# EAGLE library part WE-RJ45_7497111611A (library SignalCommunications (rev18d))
Order Code 7497111611A Design THT xBase-T 10/100/1000 Base-T Ports 1x1 + 2xUSB Application Standard USB2.0 Tab Position UP LED (Left-Right) GREEN/ORANGE-YELLOW EMI Fingers YES Details see: http://katalog.we-online.de/en/pbs/WE-LAN_RJ45/7497111611A? Updated by Yingchun Shan 2016-08-23 2014 (C) Würth Elektronik
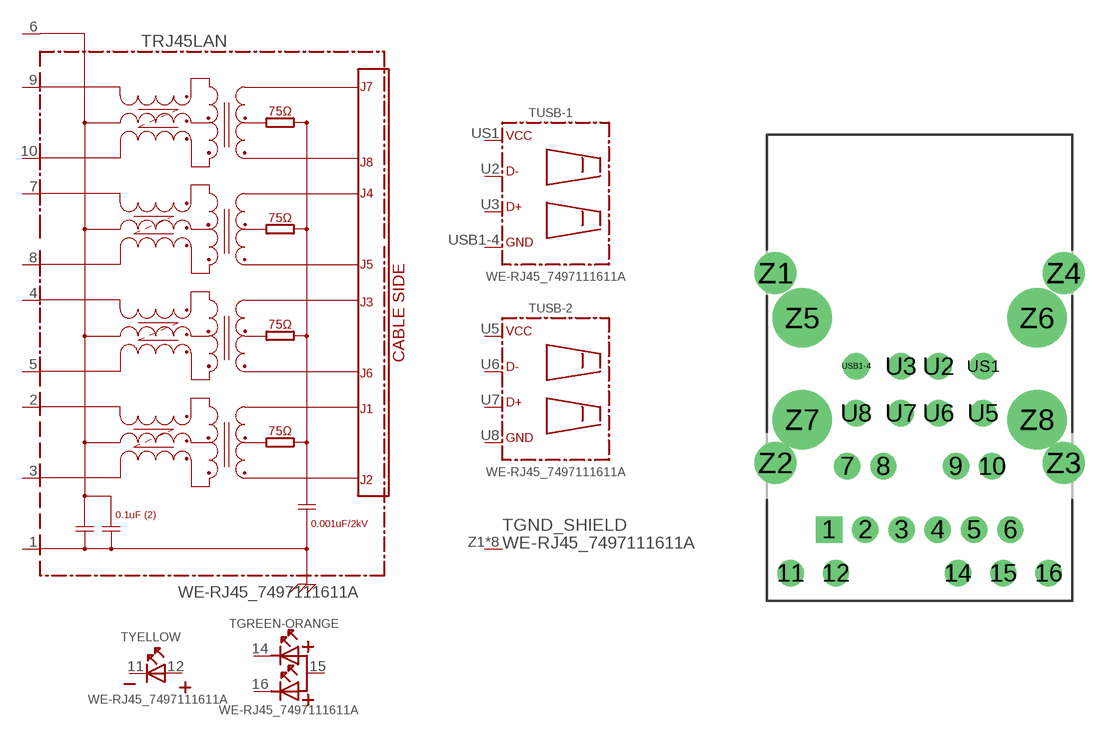
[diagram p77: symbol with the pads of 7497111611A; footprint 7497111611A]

Designator prefix T; gates RJ45LAN=7497111611A USB-1=USB2.0 USB-2=USB2.0 GND_SHIELD=GND_PIN YELLOW=LED-2PIN GREEN-ORANGE=LED-DUAL1

## WE-RJ45_7497111611A (COMPANY-URL: http://www.we-online.de; CREATED-BY: Christin Zierenner; CREATED-DATE: AUG 2012; DATASHEET-URL: http://katalog.we-online.de/kataloge/eisos/media/pdf/7497111611A.pdf; MANUFACTURER: Würth Elektronik eiSos GmbH)  [7497111611A]
1  RJ45LAN:1  pwr
2  RJ45LAN:2
3  RJ45LAN:3
4  RJ45LAN:4
5  RJ45LAN:5
6  RJ45LAN:6
7  RJ45LAN:7
8  RJ45LAN:8
9  RJ45LAN:9
10  RJ45LAN:10
11  YELLOW:K  pas
12  YELLOW:A  pas
14  GREEN-ORANGE:K1  pas
15  GREEN-ORANGE:A1  pas
16  GREEN-ORANGE:K2  pas
U2  USB-1:D-
U3  USB-1:D+
U5  USB-2:VCC  pwr
U6  USB-2:D-
U7  USB-2:D+
U8  USB-2:GND  pwr
US1  USB-1:VCC  pwr
USB1-4  USB-1:GND  pwr
Z1  GND_SHIELD:1  pwr
Z2  GND_SHIELD:1  pwr
Z3  GND_SHIELD:1  pwr
Z4  GND_SHIELD:1  pwr
Z5  GND_SHIELD:1  pwr
Z6  GND_SHIELD:1  pwr
Z7  GND_SHIELD:1  pwr
Z8  GND_SHIELD:1  pwr

## Footprint 7497111611A (pad centres in mm)
MAX HEIGHT=13.50mm PORTS----1X1 + 2XUSB (USB2.0) LED -YES
drill 0.97 square: 1 -5.075,-14.35
drill 0.97: 2 -3.045,-14.35; 3 -1.015,-14.35; 4 1.015,-14.35; 5 3.045,-14.35; 6 5.075,-14.35; 7 -4.06,-10.8; 8 -2.03,-10.8; 9 2.03,-10.8; 10 4.06,-10.8; 11 -7.225,-16.78; 12 -4.685,-16.78; 14 2.145,-16.78; 15 4.685,-16.78; 16 7.225,-16.78; U2 1.05,-5.21; U3 -1.05,-5.21; U5 3.55,-7.83; U6 1.05,-7.83; U7 -1.05,-7.83; U8 -3.55,-7.83; US1 3.55,-5.21; USB1-4 -3.55,-5.21
drill 1.57: Z1 -8.065,0; Z4 8.065,0
drill 1.57 pad 2.3: Z2 -8.065,-10.62; Z3 8.065,-10.62
drill 2.31: Z5 -6.565,-2.51; Z6 6.565,-2.51
drill 2.31 pad 3.2: Z7 -6.565,-8.2; Z8 6.565,-8.2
